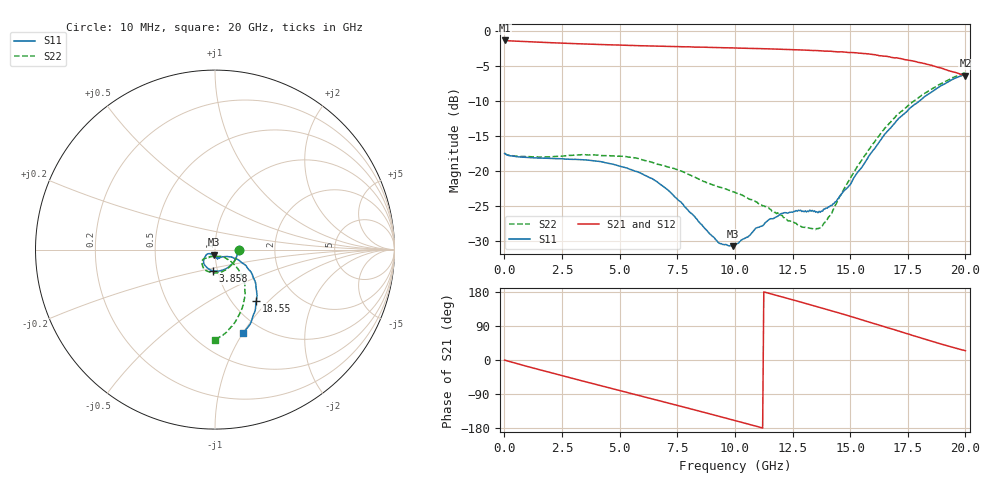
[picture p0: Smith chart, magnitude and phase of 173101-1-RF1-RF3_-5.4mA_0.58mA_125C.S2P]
!  2-Port S-parameters saved by WinCal
! VAR MeasName=S-Parameters (CALIBRATED_DATA) read from VNA (N5242A)
! VAR MeasDate=2017-7-20 10:53:57
! VAR NAME=173101-1-RF1-RF3_-5.4mA_0.58mA_125C
! VAR FILENAME=173101-1-RF1-RF3_-5.4mA_0.58mA_125C.S2P
! VAR DATE=2017-7-20 10:53:57
! VAR PHYS_PORTS=1,2
# Hz S DB R 50
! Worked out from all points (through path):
!   401 points, 10 MHz to 20 GHz, reference 50 ohm
!   highest |S21| = -1.37 dB at 10 MHz (marker M1); lowest = -6.4 dB at 20 GHz (marker M2)
!   group delay of S21, straight-line fit = 46.2 ps
!   lowest |S11| = -30.7 dB at 9.905 GHz (marker M3), VSWR 1.06, Z = 49.3 - j2.82 ohm
!   |S11| at or under -10 dB: start of sweep to 18.01 GHz
!   |S22| runs from -28.3 to -6.0 dB; largest |S21 - S12| = 0.0062
!   S11 on the Smith chart (normalised r, x): 10 MHz: 1.31, -0.01; 3.858 GHz: 0.95, -0.23; 18.55 GHz: 1.28, -0.85; 20 GHz: 0.82, -1.01
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1e7  -17.49 -1.0  -1.37 -0.2  -1.37 -0.2  -17.46 -0.8
1.559225e9  -18.15 -44.7  -1.62 -26.3  -1.63 -26.3  -17.99 -44.0
2.50875e9  -18.25 -67.9  -1.75 -41.5  -1.76 -41.4  -17.87 -66.4
3.358325e9  -18.39 -86.7  -1.87 -54.9  -1.87 -54.9  -17.66 -83.5
3.858075e9  -18.53 -96.0  -1.92 -62.7  -1.93 -62.7  -17.69 -92.1
5.30735e9  -19.55 -122.2  -2.07 -85.3  -2.08 -85.4  -17.95 -114.6
6.70665e9  -21.74 -138.6  -2.18 -107.3  -2.18 -107.3  -19.06 -129.0
7.956025e9  -25.53 -149.4  -2.28 -127.0  -2.30 -127.0  -20.41 -138.6
9.255375e9  -30.11 -128.6  -2.38 -147.8  -2.38 -147.7  -22.22 -139.9
9.90505e9  -30.71 -101.5  -2.43 -158.2  -2.44 -158.3  -22.93 -137.6
1.0005e10  -30.53 -98.5  -2.45 -159.8  -2.46 -159.9  -23.04 -137.3
1.090455e10  -28.15 -81.0  -2.52 -174.5  -2.53 -174.4  -24.36 -130.4
1.165418e10  -26.80 -78.5  -2.59 173.1  -2.60 173.1  -25.73 -127.0
1.210395e10  -26.00 -76.5  -2.63 165.7  -2.64 165.7  -26.60 -123.3
1.335332e10  -25.61 -66.4  -2.80 144.4  -2.78 144.5  -28.20 -90.6
1.375312e10  -25.70 -57.4  -2.86 137.4  -2.86 137.4  -27.81 -70.1
1.430285e10  -24.62 -42.3  -2.96 127.8  -2.97 127.9  -25.29 -46.2
1.545228e10  -19.68 -23.9  -3.19 107.0  -3.21 106.9  -18.70 -37.1
1.670165e10  -14.01 -28.0  -3.70 83.7  -3.76 83.5  -13.18 -45.3
1.76012e10  -11.00 -37.8  -4.22 67.2  -4.22 67.2  -10.40 -56.1
1.855072e10  -8.69 -51.2  -4.93 49.2  -5.00 49.4  -8.28 -69.4
2e10  -6.15 -71.4  -6.40 24.5  -6.45 25.0  -5.96 -89.9
